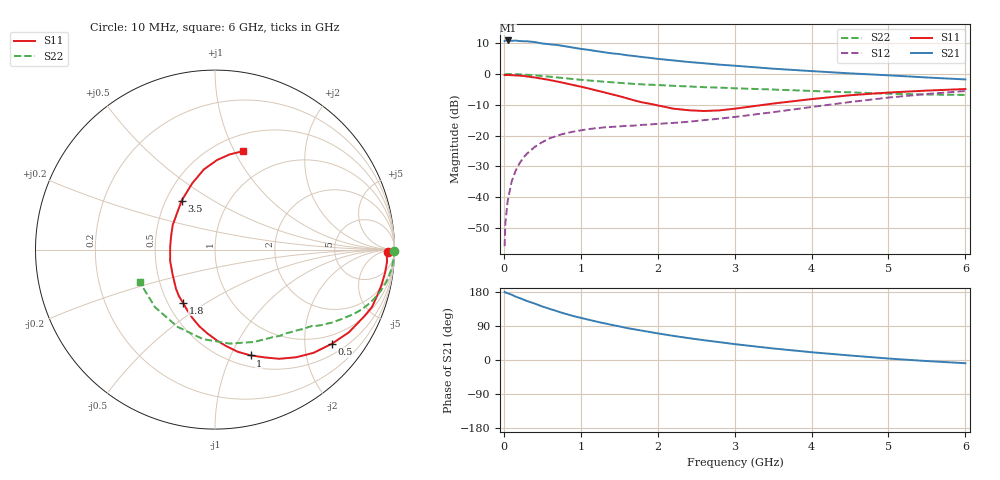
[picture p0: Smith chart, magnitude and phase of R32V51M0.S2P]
! SIEMENS Small Signal Semiconductors
! BFR181
! Si NPN RF Bipolar Junction Transistor in SOT23
! VCE = 2.5 V  IC = 1 mA
! Common Emitter S-Parameters:  May  1996
# GHz  S  MA  R  50
!  f  S11  S21  S12  S22
! GHz  MAG  ANG  MAG  ANG  MAG  ANG  MAG  ANG
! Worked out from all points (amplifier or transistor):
!   36 points, 10 MHz to 6 GHz, reference 50 ohm
!   highest |S21| = 10.9 dB at 50 MHz (marker M1)
!   |S21| within 3 dB of that: start of sweep to 1.084 GHz
!   unconditionally stable (mu >= 1): 2.006 GHz to 3.667 GHz
!   at 250 MHz: K = 0.16, MSG = 18.9 dB, |S12| = -27.3 dB
!   at 1.4 GHz: K = 0.77, MSG = 12.0 dB, |S12| = -17.2 dB
!   at 6 GHz: K = 0.88, MSG = 1.9 dB, |S12| = -5.5 dB
!   lowest NFmin = 1.30 dB at 450 MHz
!   S11 on the Smith chart (normalised r, x): 10 MHz: 45, -18; 500 MHz: 0.76, -2.64; 1 GHz: 0.62, -1.19; 1.8 GHz: 0.60, -0.40; 3.5 GHz: 0.60, +0.37; 6 GHz: 0.67, +1.08
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0.01  0.9622 -0.9  3.426 179.5  0.0016 94.2  0.999 -0.4
0.02  0.9573 -1.4  3.476 178.3  0.0038 95.7  0.9876 -0.7
0.05  0.9609 -4.0  3.498 176.1  0.0087 85.3  0.9976 -1.9
0.1  0.9562 -7.9  3.442 172.4  0.0176 86.1  0.9948 -3.8
0.15  0.9484 -12.0  3.486 167.5  0.0263 81.3  0.99 -5.8
0.2  0.9396 -15.8  3.427 163.9  0.0347 79.2  0.9839 -7.5
0.3  0.9109 -24.1  3.39 155.7  0.0508 74.8  0.9698 -11.0
0.4  0.8769 -31.7  3.3 149.0  0.0651 69.7  0.9492 -14.4
0.5  0.836 -38.9  3.121 141.2  0.0783 65.8  0.9264 -17.4
0.7  0.7511 -53.0  2.942 128.2  0.1002 58.5  0.8768 -22.7
0.8  0.7061 -59.5  2.812 121.9  0.1087 55.0  0.8511 -25.0
1  0.6221 -71.4  2.555 111.3  0.1214 50.3  0.8039 -28.8
1.1  0.5828 -77.5  2.462 106.4  0.1272 48.6  0.7852 -30.4
1.4  0.4684 -95.3  2.164 92.8  0.1381 44.6  0.7333 -34.9
1.6  0.4027 -108.0  2.012 84.3  0.1438 43.5  0.704 -37.2
1.8  0.3452 -121.2  1.88 77.3  0.1491 43.8  0.6778 -39.4
2.2  0.2736 -149.8  1.66 63.8  0.1602 45.3  0.642 -44.5
3  0.2727 149.7  1.361 41.9  0.2003 50.2  0.585 -56.5
3.5  0.3305 124.2  1.218 30.5  0.2397 51.4  0.5587 -67.1
4.5  0.451 97.9  1.022 11.9  0.3499 46.9  0.5033 -97.6
5.5  0.5369 81.2  0.876 -2.8  0.4732 34.3  0.4633 -136.2
6  0.5692 74.3  0.815 -8.5  0.5281 26.5  0.4569 -156.6
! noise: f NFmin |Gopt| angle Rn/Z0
0.45  1.3  0.7  18  0.5
0.9  1.4  0.6  39  0.52
1.8  1.85  0.4  81  0.47
